|   IBIS file stm32l476_wlcsp81.ibs
[IBIS ver]   4.2
[File name]   stm32l476_wlcsp81.ibs
[File Rev]   4.0
[Date]   08-10-2018
[Source]   Data Created at STMicroelectronics
[Notes]   File originated from ELDO simulations.
[Disclaimer]  This information is for modeling purpose only and is
   not guaranteed.
   The information is subject to change without notice.
[Copyright]   Copyright 2018 STMicroelectronics Inc.
|   Component stm32l476_wlcsp81
[Component] stm32l476_wlcsp81
[Manufacturer] STMicroelectronics
[Package]
| variable   typ   min   max
R_pkg   0.0   0.0   0.0
L_pkg   0.0H   0.0H   0.0H
C_pkg   0.0F   0.0F   0.0F
[Pin]  signal_name   model_name   R_pin   L_pin   C_pin
A1 VDDUSB POWER
A2 PA15 io8prog2m25m50m120m_sudq_ft
A3 PD2 io8prog2m25m50m120m_sudq_ft
A4 PG9 io8prog2m25m50m120m_sudq_ft
A5 PG14 io8prog2m25m50m120m_sudq_i2c_ft
A6 PB3 io8prog2m25m50m120m_sudq_ft
A7 PB7 io8prog2m25m50m120m_sudq_i2c_ft
A8 VSS GND
A9 VDD POWER
B1 VSS GND
B2 PA14 io8prog2m25m50m120m_sudq_ft
B3 PC12 io8prog2m25m50m120m_sudq_ft
B4 PG10 io8prog2m25m50m120m_sudq_ft
B5 PG13 io8prog2m25m50m120m_sudq_i2c_ft
B6 VDDIO2 POWER
B7 PB6 io8prog2m25m50m120m_sudq_i2c_ft
B8 PC13 io8prog2m25m50m120m_sudq_ft
B9 VBAT POWER
C1 PA12 io8usblsfs_otg2
C2 PA13 io8prog2m25m50m120m_sudq_ft
C3 PC11 io8prog2m25m50m120m_sudq_ft
C4 PG11 io8prog2m25m50m120m_sudq_ft
C5 PG12 io8prog2m25m50m120m_sudq_ft
C6 PB4 io8prog2m25m50m120m_sudq_ft
C7 PB5 io8prog2m25m50m120m_sudq_ft
C8 PC15-OSC32_OUT io8prog2m25m50m120m_sudq_ft
C9 PC14-OSC32_IN io8prog2m25m50m120m_sudq_ft
D1 PA11 io8usblsfs_otg2
D2 PA10 io8usb_id_otg20_lcd4_ft_ms
D3 PC10 io8prog2m25m50m120m_sudq_ft
D4 PD5 io8prog2m25m50m120m_sudq_ft
D5 PD6 io8prog2m25m50m120m_sudq_ft
D6 PD7 io8prog2m25m50m120m_sudq_ft
D7 BOOT0 vpp_test_hv
D8 PH1-OSC_OUT io8prog2m25m50m120m_sudq_ft
D9 PH0-OSC_IN io8prog2m25m50m120m_sudq_ft
E1 PC9 io8prog2m25m50m120m_sudq_ft
E2 PA8 io8prog2m25m50m120m_sudq_ft
E3 PA9 POWER
E4 VDD POWER
E5 PD4 io8prog2m25m50m120m_sudq_ft
E6 PE7 io8prog2m25m50m120m_sudq_ft
E7 PB8 io8prog2m25m50m120m_sudq_i2c_ft
E8 PB9 io8prog2m25m50m120m_sudq_i2c_ft
E9 NRST ioreset_ft_v33
F1 PC7 io8prog2m25m50m120m_sudq_ft
F2 PC8 io8prog2m25m50m120m_sudq_ft
F3 PC6 io8prog2m25m50m120m_sudq_ft
F4 PD9 io8prog2m25m50m120m_sudq_ft
F5 PD8 io8prog2m25m50m120m_sudq_ft
F6 PE8 io8prog2m25m50m120m_sudq_ft
F7 PC2 io8prog2m25m50m120m_sudq_ft
F8 PC1 io8prog2m25m50m120m_sudq_i2c_ft
F9 PC0 io8prog2m25m50m120m_sudq_i2c_ft
G1 PB15 io8prog2m25m50m120m_sudq_ft
G2 PB14 io8prog2m25m50m120m_sudq_i2c_ft
G3 PB11 io8prog2m25m50m120m_sudq_i2c_ft
G4 PA1 io8prog2m25m50m120m_sudq_ft
G5 PA4 io8prog2m25m50m120m_sudq_ft
G6 PA2 io8prog2m25m50m120m_sudq_ft
G7 PC3 io8prog2m25m50m120m_sudq_ft
G8 VREF+ POWER
G9 VSSA_VREF- GND
H1 PB12 io8w_swp_lcd4_ft
H2 PB13 io8prog2m25m50m120m_sudq_i2c_ft
H3 PB10 io8prog2m25m50m120m_sudq_i2c_ft
H4 PA7 io8prog2m25m50m120m_sudq_ft
H5 PA6 io8prog2m25m50m120m_sudq_ft
H6 PA5 io8prog2m25m50m120m_sudq_ft
H7 PA3 io8prog2m25m50m120m_sudq_ft
H8 PA0 io8prog2m25m50m120m_sudq_ft
H9 VDDA POWER
J1 VDD POWER
J2 VSS GND
J3 PB2 io8prog2m25m50m120m_sudq_ft
J4 PB1 io8prog2m25m50m120m_sudq_ft
J5 PB0 io8prog2m25m50m120m_sudq_ft
J6 PC5 io8prog2m25m50m120m_sudq_ft
J7 PC4 io8prog2m25m50m120m_sudq_ft
J8 VDD POWER
J9 VSS GND
[Model Selector] io8prog2m25m50m120m_sudq_ft
iols8p_sudq_ft_pd_lv  "IO low speed, PD=40kOhm - 1P8V"
iols8p_sudq_ft_pu_lv  "IO low speed, PU=40kOhm - 1P8V"
iols8p_sudq_ft_lv  "IO low speed - 1P8V"
iols8p_sudq_ft_pd  "IO low speed, PD=40kOhm - 3P3V"
iols8p_sudq_ft_pu  "IO low speed, PU=40kOhm - 3P3V"
iols8p_sudq_ft  "IO low speed - 3P3V"
iofs8p_sudq_ft_pd_lv  "IO full speed, PD=40kOhm - 1P8V"
iofs8p_sudq_ft_pu_lv  "IO full speed, PU=40kOhm - 1P8V"
iofs8p_sudq_ft_lv  "IO full speed - 1P8V"
iofs8p_sudq_ft_pd  "IO full speed, PD=40kOhm - 3P3V"
iofs8p_sudq_ft_pu  "IO full speed, PU=40kOhm - 3P3V"
iofs8p_sudq_ft  "IO full speed - 3P3V"
ioms8p_sudq_ft_pd_lv  "IO medium speed, PD=40kOhm - 1P8V"
ioms8p_sudq_ft_pu_lv  "IO medium speed, PU=40kOhm - 1P8V"
ioms8p_sudq_ft_lv  "IO medium speed - 1P8V"
ioms8p_sudq_ft_pd  "IO medium speed, PD=40kOhm - 3P3V"
ioms8p_sudq_ft_pu  "IO medium speed, PU=40kOhm - 3P3V"
ioms8p_sudq_ft  "IO medium speed - 3P3V"
iohs8p_sudq_ft_pd_lv  "IO high speed, PD=40kOhm - 1P8V"
iohs8p_sudq_ft_pu_lv  "IO high speed, PU=40kOhm - 1P8V"
iohs8p_sudq_ft_lv  "IO high speed - 1P8V"
iohs8p_sudq_ft_pd  "IO high speed, PD=40kOhm - 3P3V"
iohs8p_sudq_ft_pu  "IO high speed, PU=40kOhm - 3P3V"
iohs8p_sudq_ft  "IO high speed - 3P3V"
[Model Selector] io8prog2m25m50m120m_sudq_i2c_ft
io8prog_1v8_i2c_pd  "5V Tol GPIO 1.8V range i2c functionality with pull down"
io8prog_1v8_i2c_pu  "5V Tol GPIO 1.8V range i2c functionality with pull up"
io8prog_1v8_i2c  "5V Tol GPIO 1.8V range i2c functionality"
io8prog_3v3_i2c_pd  "5V Tol GPIO 3.3V range i2c functionality with pull down"
io8prog_3v3_i2c_pu  "5V Tol GPIO 3.3V range i2c functionality with pull up"
io8prog_3v3_i2c  "5V Tol GPIO 3.3V range i2c functionality"
io8ls_1v8_pd  "5V Tol GPIO 1.8V range with pd io low speed"
io8ls_1v8_pu  "5V Tol GPIO 1.8V range with pu io low speed"
io8ls_1v8  "5V Tol GPIO 1.8V range io low speed"
io8ls_3v3_pd  "5V Tol GPIO 3.3V range with pd io low speed"
io8ls_3v3_pu  "5V Tol GPIO 3.3V range with pu io low speed"
io8ls_3v3  "5V Tol GPIO 3.3V range io low speed"
io8fs_1v8_pd  "5V Tol GPIO 1.8V range with pd io full speed"
io8fs_1v8_pu  "5V Tol GPIO 1.8V range with pu io full speed"
io8fs_1v8  "5V Tol GPIO 1.8V range io full speed"
io8fs_3v3_pd  "5V Tol GPIO 3.3V range with pd io full speed"
io8fs_3v3_pu  "5V Tol GPIO 3.3V range with pu io full speed"
io8fs_3v3  "5V Tol GPIO 3.3V range io full speed"
io8ms_1v8_pd  "5V Tol GPIO 1.8V range with pd io medium speed"
io8ms_1v8_pu  "5V Tol GPIO 1.8V range with pu io medium speed"
io8ms_1v8  "5V Tol GPIO 1.8V range io medium speed"
io8ms_3v3_pd  "5V Tol GPIO 3.3V range with pd io medium speed"
io8ms_3v3_pu  "5V Tol GPIO 3.3V range with pu io medium speed"
io8ms_3v3  "5V Tol GPIO 3.3V range io medium speed"
io8hs_1v8_pd  "5V Tol GPIO 1.8V range with pd io high speed"
io8hs_1v8_pu  "5V Tol GPIO 1.8V range with pu io high speed"
io8hs_1v8  "5V Tol GPIO 1.8V range io high speed"
io8hs_3v3_pd  "5V Tol GPIO 3.3V range with pd io high speed"
io8hs_3v3_pu  "5V Tol GPIO 3.3V range with pu io high speed"
io8hs_3v3  "5V Tol GPIO 3.3V range io high speed"
[Model Selector] io8usb_id_otg20_lcd4_ft_ms
io8usbid_1v8_id_pu  "ID 1V8 range with pull up"
io8usbid_3v3_id_pu  "ID 3V3 range with pull up"
io8usbid_1v8_id  "ID 1V8 range"
io8usbid_3v3_id  "ID 3V3 range"
io8lsusbid_1v8_pd  "GPIO 1.8V range with pd io low speed"
io8lsusbid_1v8_pu  "GPIO 1.8V range with pu io low speed"
io8lsusbid_1v8  "GPIO 1.8V range io low speed"
io8lsusbid_3v3_pd  "GPIO 3.3V range with pd io low speed"
io8lsusbid_3v3_pu  "GPIO 3.3V range with pu io low speed"
io8lsusbid_3v3  "GPIO 3.3V range io low speed"
io8fsusbid_1v8_pd  "GPIO 1.8V range with pd io full speed"
io8fsusbid_1v8_pu  "GPIO 1.8V range with pu io full speed"
io8fsusbid_1v8  "GPIO 1.8V range io full speed"
io8fsusbid_3v3_pd  "GPIO 3.3V range with pd io full speed"
io8fsusbid_3v3_pu  "GPIO 3.3V range with pu io full speed"
io8fsusbid_3v3  "GPIO 3.3V range io full speed"
io8msusbid_1v8_pd  "GPIO 1.8V range with pd io medium speed"
io8msusbid_1v8_pu  "GPIO 1.8V range with pu io medium speed"
io8msusbid_1v8  "GPIO 1.8V range io medium speed"
io8msusbid_3v3_pd  "GPIO 3.3V range with pd io medium speed"
io8msusbid_3v3_pu  "GPIO 3.3V range with pu io medium speed"
io8msusbid_3v3  "GPIO 3.3V range io medium speed"
io8hsusbid_1v8_pd  "GPIO 1.8V range with pd io high speed"
io8hsusbid_1v8_pu  "GPIO 1.8V range with pu io high speed"
io8hsusbid_1v8  "GPIO 1.8V range io high speed"
io8hsusbid_3v3_pd  "GPIO 3.3V range with pd io high speed"
io8hsusbid_3v3_pu  "GPIO 3.3V range with pu io high speed"
io8hsusbid_3v3  "GPIO 3.3V range io high speed"
[Model Selector] io8usblsfs_otg2
usb_ls_pd  "USB Low Speed mode - Pull Down"
usb_ls_pu2  "USB Low Speed mode - Pull up 2"
usb_ls_pu  "USB Low Speed mode - Pull up"
usb_fs  "USB Low Speed mode"
usb_fs_pd  "USB Full Speed mode - Pull Down"
usb_fs_pu2  "USB Full Speed mode - Pull up 2"
usb_fs_pu  "USB Full Speed mode - Pull up"
[Model Selector] ioreset_ft_v33
ioreset_1v2_pu  "RESET 1.2V range with PU"
ioreset_1v2  "RESET 1.2V range"
ioreset_1v8_pu  "RESET 1.8V range with PU"
ioreset_1v8  "RESET 1.8V range"
ioreset_3v3_pu  "RESET 3.3V range with PU"
ioreset_3v3  "RESET 3.3V range"
[Model Selector] io8w_swp_lcd4_ft
io8w_swp_classc  "Class C swp functionality"
io8w_swp_classb  "Class B swp functionality"
io8lsw_1v8_pd  "GPIO 1.8V range with pd io low speed"
io8lsw_1v8_pu  "GPIO 1.8V range with pu io low speed"
io8lsw_1v8  "GPIO 1.8V range io low speed"
io8lsw_3v3_pd  "GPIO 3.3V range with pd io low speed"
io8lsw_3v3_pu  "GPIO 3.3V range with pu io low speed"
io8lsw_3v3  "GPIO 3.3V range io low speed"
io8fsw_1v8_pd  "GPIO 1.8V range with pd io full speed"
io8fsw_1v8_pu  "GPIO 1.8V range with pu io full speed"
io8fsw_1v8  "GPIO 1.8V range io full speed"
io8fsw_3v3_pd  "GPIO 3.3V range with pd io full speed"
io8fsw_3v3_pu  "GPIO 3.3V range with pu io full speed"
io8fsw_3v3  "GPIO 3.3V range io full speed"
io8msw_1v8_pd  "GPIO 1.8V range with pd io medium speed"
io8msw_1v8_pu  "GPIO 1.8V range with pu io medium speed"
io8msw_1v8  "GPIO 1.8V range io medium speed"
io8msw_3v3_pd  "GPIO 3.3V range with pd io medium speed"
io8msw_3v3_pu  "GPIO 3.3V range with pu io medium speed"
io8msw_3v3  "GPIO 3.3V range io medium speed"
io8hsw_1v8_pd  "GPIO 1.8V range with pd io high speed"
io8hsw_1v8_pu  "GPIO 1.8V range with pu io high speed"
io8hsw_1v8  "GPIO 1.8V range io high speed"
io8hsw_3v3_pd  "GPIO 3.3V range with pd io high speed"
io8hsw_3v3_pu  "GPIO 3.3V range with pu io high speed"
io8hsw_3v3  "GPIO 3.3V range io high speed"
[Model Selector] vpp_test_hv
vpp_1v8  "VPP with test functionality 1.8V range"
vpp_3v3  "VPP with test functionality 3.3V range"
| Models and submodels in the file (123): iols8p_sudq_ft_pd_lv (I/O), iols8p_sudq_ft_pu_lv (I/O), iols8p_sudq_ft_lv (I/O), iols8p_sudq_ft_pd (I/O), iols8p_sudq_ft_pu (I/O), iols8p_sudq_ft (I/O), iofs8p_sudq_ft_pd_lv (I/O), iofs8p_sudq_ft_pu_lv (I/O), iofs8p_sudq_ft_lv (I/O), iofs8p_sudq_ft_pd (I/O), iofs8p_sudq_ft_pu (I/O), iofs8p_sudq_ft (I/O), ioms8p_sudq_ft_pd_lv (I/O), ioms8p_sudq_ft_pu_lv (I/O), ioms8p_sudq_ft_lv (I/O), ioms8p_sudq_ft_pd (I/O), ioms8p_sudq_ft_pu (I/O), ioms8p_sudq_ft (I/O), iohs8p_sudq_ft_pd_lv (I/O), iohs8p_sudq_ft_pu_lv (I/O), iohs8p_sudq_ft_lv (I/O), iohs8p_sudq_ft_pd (I/O), iohs8p_sudq_ft_pu (I/O), iohs8p_sudq_ft (I/O), io8prog_1v8_i2c_pd (I/O), io8prog_1v8_i2c_pu (I/O), io8prog_1v8_i2c (I/O), io8prog_3v3_i2c_pd (I/O), io8prog_3v3_i2c_pu (I/O), io8prog_3v3_i2c (I/O), io8ls_1v8_pd (I/O), io8ls_1v8_pu (I/O), io8ls_1v8 (I/O), io8ls_3v3_pd (I/O), io8ls_3v3_pu (I/O), io8ls_3v3 (I/O), io8fs_1v8_pd (I/O), io8fs_1v8_pu (I/O), io8fs_1v8 (I/O), io8fs_3v3_pd (I/O), io8fs_3v3_pu (I/O), io8fs_3v3 (I/O), io8ms_1v8_pd (I/O), io8ms_1v8_pu (I/O), io8ms_1v8 (I/O), io8ms_3v3_pd (I/O), io8ms_3v3_pu (I/O), io8ms_3v3 (I/O), io8hs_1v8_pd (I/O), io8hs_1v8_pu (I/O), io8hs_1v8 (I/O), io8hs_3v3_pd (I/O), io8hs_3v3_pu (I/O), io8hs_3v3 (I/O), io8usbid_1v8_id_pu (Input), io8usbid_3v3_id_pu (Input), io8usbid_1v8_id (Input), io8usbid_3v3_id (Input), io8lsusbid_1v8_pd (I/O), io8lsusbid_1v8_pu (I/O), io8lsusbid_1v8 (I/O), io8lsusbid_3v3_pd (I/O), io8lsusbid_3v3_pu (I/O), io8lsusbid_3v3 (I/O), io8fsusbid_1v8_pd (I/O), io8fsusbid_1v8_pu (I/O), io8fsusbid_1v8 (I/O), io8fsusbid_3v3_pd (I/O), io8fsusbid_3v3_pu (I/O), io8fsusbid_3v3 (I/O), io8msusbid_1v8_pd (I/O), io8msusbid_1v8_pu (I/O), io8msusbid_1v8 (I/O), io8msusbid_3v3_pd (I/O), io8msusbid_3v3_pu (I/O), io8msusbid_3v3 (I/O), io8hsusbid_1v8_pd (I/O), io8hsusbid_1v8_pu (I/O), io8hsusbid_1v8 (I/O), io8hsusbid_3v3_pd (I/O)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
